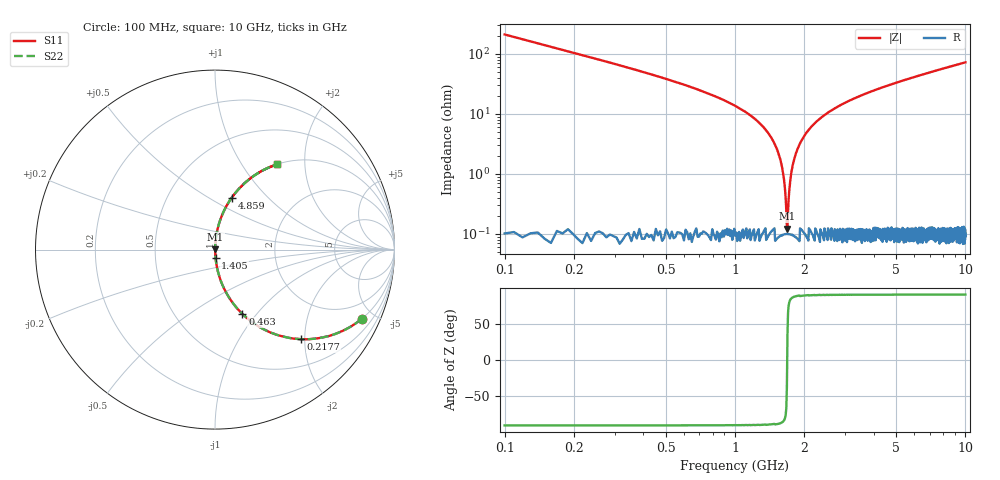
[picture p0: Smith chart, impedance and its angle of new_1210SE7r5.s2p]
!	AVX	Thin	Film	Operation	Date:	April 2007
!	Description:	Accu-P®	"Series,"	Thin	"Film,"	"SMD,"	RF	Capacitor
!	Part	Number:	12101J7R5BBT
!	100	MHz	-	5.05	GHz
!	Serial	Measurements
#	MHZ	S	MA	R	50
!	S11	S21	S12	S22
!	dB	Phase	dB	Phase	dB	Phase	dB	Phase
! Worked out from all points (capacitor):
!   1010 points, 100 MHz to 10 GHz, reference 50 ohm
!   read as one part in series: C = 7.5 pF near 149.1 MHz
!   lowest |Z| = 122 mohm at 1.689 GHz (marker M1)
!   series resonance near 1.685 GHz, so ESL is about 1.2 nH
!   S11 on the Smith chart (normalised r, x): 100 MHz: 1.00, -4.23; 217.7 MHz: 1.00, -1.92; 463 MHz: 1.00, -0.85; 1.405 GHz: 1.00, -0.09; 4.859 GHz: 1.00, +0.64; 10 GHz: 1.00, +1.45
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100  0.904 -25.3  0.427 64.7  0.427 64.7  0.904 -25.3
217.74  0.692 -46.2  0.722 43.8  0.722 43.8  0.692 -46.2
325.669  0.531 -57.8  0.847 32.1  0.847 32.1  0.531 -57.8
463.033  0.39 -66.9  0.92 22.9  0.92 22.9  0.39 -66.9
1120.416  0.105 -83.4  0.993 6.0  0.993 6.0  0.105 -83.4
1404.955  0.046 -86.1  0.998 2.6  0.998 2.6  0.046 -86.1
1552.131  0.021 -86.0  0.999 1.2  0.999 1.2  0.021 -86.0
1601.189  0.013 -84.8  0.999 0.7  0.999 0.7  0.013 -84.8
1650.248  0.00531 -78.8  0.999 0.3  0.999 0.3  0.00531 -78.8
1689.495  0.00122 35.1  0.999 -0.0  0.999 -0.0  0.00122 35.1
1718.93  0.00515 78.5  0.999 -0.3  0.999 -0.3  0.00515 78.5
1758.176  0.011 84.1  0.999 -0.6  0.999 -0.6  0.011 84.1
1807.235  0.018 85.8  0.999 -1.0  0.999 -1.0  0.018 85.8
1895.54  0.03 86.4  0.999 -1.7  0.999 -1.7  0.03 86.4
2180.079  0.065 85.4  0.997 -3.8  0.997 -3.8  0.065 85.4
2660.852  0.118 82.7  0.992 -6.8  0.992 -6.8  0.118 82.7
3406.541  0.189 78.8  0.981 -10.9  0.981 -10.9  0.189 78.8
4858.672  0.304 72.1  0.952 -17.7  0.952 -17.7  0.304 72.1
5054.906  0.318 71.3  0.947 -18.6  0.947 -18.6  0.318 71.3
6703.271  0.425 64.8  0.904 -25.1  0.904 -25.1  0.425 64.8
8351.635  0.513 59.0  0.857 -30.9  0.857 -30.9  0.513 59.0
10000  0.587 54.0  0.809 -36.0  0.809 -36.0  0.587 54.0
